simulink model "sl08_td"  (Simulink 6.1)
settings: Solver=ode45  StartTime=0.0  StopTime=0.1  MaxStep=0.001  RelTol=1e-3
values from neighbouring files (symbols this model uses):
  G1den = [0.05 15.008 2.4]    [sl08.m]
  G1num = 1.5    [sl08.m]
  G2den = [6.25 1]    [sl08.m]
  G2num = 12.5    [sl08.m]
undefined symbols (not defined in the file or in its folder): Rzden, Rznum

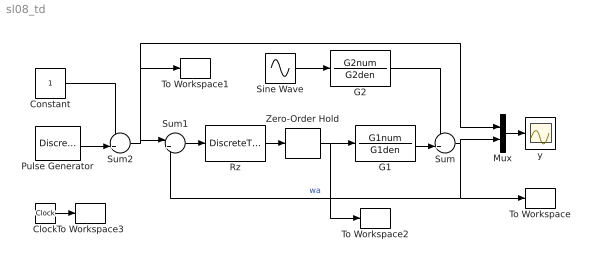
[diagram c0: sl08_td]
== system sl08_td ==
  Clock : Clock
  Constant : Constant  Value=1
  G1 : TransferFcn  Numerator=G1num  Denominator=G1den  AbsoluteTolerance=auto  Realization=auto
  G2 : TransferFcn  Numerator=G2num  Denominator=G2den  AbsoluteTolerance=auto  Realization=auto
  Mux : Mux  Inputs=2
  Pulse Generator : DiscretePulseGenerator  PulseType=Time-based  Amplitude=2  Period=0.2  PulseWidth=50  PhaseDelay=0
  Rz : DiscreteTransferFcn  Numerator=Rznum  Denominator=Rzden  Realization=auto
  Sine Wave : Sin  SineType=Time-based  Amplitude=0  Bias=0  Frequency=50  Phase=0  Samples=10
  Sum : Sum  Inputs=++|  SaturateOnIntegerOverflow=on
  Sum1 : Sum  Inputs=|+-  SaturateOnIntegerOverflow=on
  Sum2 : Sum  Inputs=-+|  SaturateOnIntegerOverflow=on
  To Workspace : ToWorkspace  VariableName=yd  SaveFormat=Array
  To Workspace1 : ToWorkspace  VariableName=wd  SaveFormat=Array
  To Workspace2 : ToWorkspace  VariableName=ud  SaveFormat=Array
  To Workspace3 : ToWorkspace  VariableName=td  SaveFormat=Array
  Zero-Order Hold : ZeroOrderHold
  y : Scope
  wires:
  Rz/1 -> Zero-Order Hold/1
  Sum/1 -> Mux/2, Sum1/2, To Workspace/1  "wa"
  Sum1/1 -> Rz/1
  Sine Wave/1 -> G2/1
  G1/1 -> Sum/2
  G2/1 -> Sum/1
  Sum2/1 -> Mux/1, To Workspace1/1, Sum1/1
  Mux/1 -> y/1
  Pulse Generator/1 -> Sum2/2
  Constant/1 -> Sum2/1
  Clock/1 -> To Workspace3/1
  Zero-Order Hold/1 -> G1/1, To Workspace2/1
